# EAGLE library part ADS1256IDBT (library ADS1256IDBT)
ADC Check availability
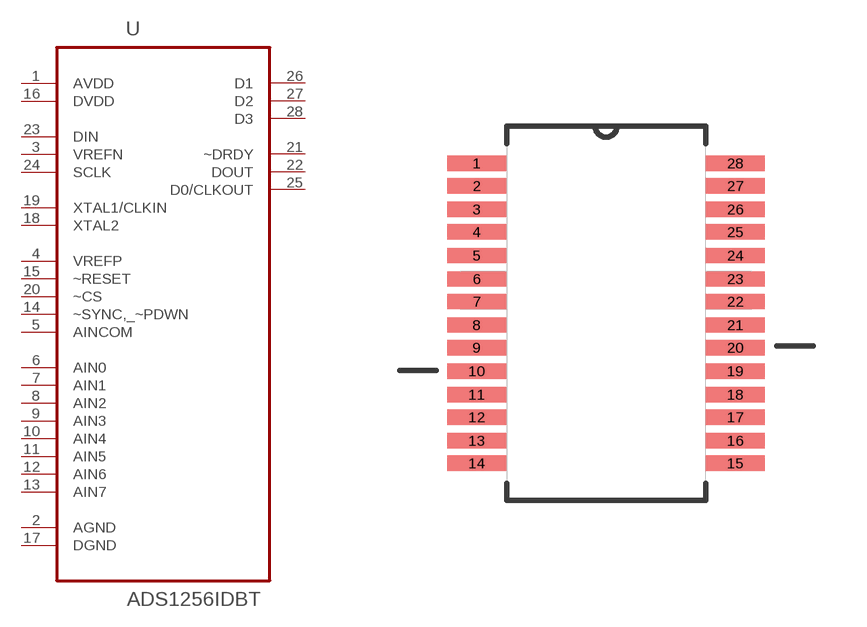
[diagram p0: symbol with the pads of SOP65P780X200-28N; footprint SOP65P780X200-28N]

Designator prefix U

## ADS1256IDBT (Availability: In Stock; Description: 24-Bit, 30kSPS, 8-Ch Delta-Sigma ADC With PGA for Factory Automation and Process Control; MF: Texas Instruments; MP: ADS1256IDBT; Package: SSOP-28 Texas Instruments; Price: None; Purchase-URL: https://pricing.snapeda.com/search/part/ADS1256IDBT/?ref=eda)  [SOP65P780X200-28N]
1  AVDD  pwr
2  AGND  pas
3  VREFN  in
4  VREFP  in
5  AINCOM  in
6  AIN0  in
7  AIN1  in
8  AIN2  in
9  AIN3  in
10  AIN4  in
11  AIN5  in
12  AIN6  in
13  AIN7  in
14  ~SYNC,_~PDWN  in
15  ~RESET  in
16  DVDD  pwr
17  DGND  pas
18  XTAL2  in
19  XTAL1/CLKIN  in
20  ~CS  in
21  ~DRDY  out
22  DOUT  out
23  DIN  in
24  SCLK  in
25  D0/CLKOUT
26  D1
27  D2
28  D3

## Footprint SOP65P780X200-28N (pad centres in mm)
smd 1.651 x 0.432: 1 -3.632,4.216; 2 -3.632,3.581; 3 -3.632,2.921; 4 -3.632,2.286; 5 -3.632,1.626; 6 -3.632,0.965; 7 -3.632,0.33; 8 -3.632,-0.33; 9 -3.632,-0.965; 10 -3.632,-1.626; 11 -3.632,-2.286; 12 -3.632,-2.921; 13 -3.632,-3.581; 14 -3.632,-4.216; 15 3.632,-4.216; 16 3.632,-3.581; 17 3.632,-2.921; 18 3.632,-2.286; 19 3.632,-1.626; 20 3.632,-0.965; 21 3.632,-0.33; 22 3.632,0.33; 23 3.632,0.965; 24 3.632,1.626; 25 3.632,2.286; 26 3.632,2.921; 27 3.632,3.581; 28 3.632,4.216

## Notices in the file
This work is licensed under a Creative Commons Attribution-ShareAlike 4.0 International License (CC BY-SA) with Design Exception 1.0
